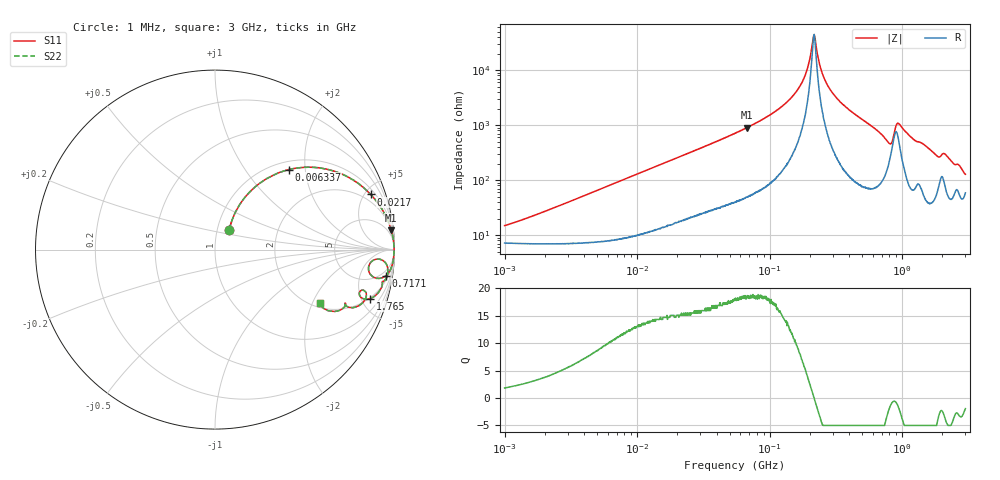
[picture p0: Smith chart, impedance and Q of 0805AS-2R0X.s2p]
!s-Parameter Generated by FASTRON Sdn. Bhd.
!FASTRON P/N : 0805AS-2R0X
!Keysight Technologies: E4991B_MY54100416_A.01.15
!Date: Mon Jun 15 12:57:28 2026
!Version  :Rev01  Mon Jun 15 12:57:28 2026
!Data & Calibration Information:
!Freq  S11  S21  S12  S22
!PortZ  Port1:50+j0  Port2:50+j0
!When reading reference impedance value at option line is always used.
! Remarks : This data is being provided solely for informational purposes.
# Hz S dB R 50
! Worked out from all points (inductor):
!   1601 points, 1 MHz to 3 GHz, reference 50 ohm
!   read as one part in series: L = 2.06 uH near 1.617 MHz
!   highest Q = 18.5 at 67.25 MHz (marker M1), where L = 2.13 uH
!   self-resonance near 215.8 MHz
!   S11 on the Smith chart (normalised r, x): 1 MHz: 1.14, +0.26; 6.337 MHz: 1.16, +1.64; 21.7 MHz: 1.36, +5.49; 717.1 MHz: 3, -13; 1.765 GHz: 1.91, -5.90; 3 GHz: 2.17, -2.27
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1000000  -17.20 54.2  -0.66 -6.9  -0.66 -6.9  -17.20 54.2
3804036  -7.49 57.0  -1.43 -24.7  -1.43 -24.7  -7.49 57.0
6337400  -4.34 47.3  -2.64 -37.2  -2.64 -37.2  -4.34 47.3
1.447069e7  -1.36 27.4  -6.71 -58.6  -6.71 -58.6  -1.36 27.4
2.170294e7  -0.72 19.5  -9.53 -66.7  -9.53 -66.7  -0.72 19.5
5.504702e7  -0.15 7.9  -17.20 -78.9  -17.20 -78.9  -0.15 7.9
6.724529e7  -0.10 6.3  -19.20 -80.6  -19.20 -80.6  -0.10 6.3
1.114693e8  -0.04 3.1  -25.20 -83.5  -25.20 -83.5  -0.04 3.1
1.543168e8  -0.03 1.5  -31.40 -82.9  -31.40 -82.9  -0.03 1.5
1.857042e8  -0.02 0.7  -38.20 -78.5  -38.20 -78.5  -0.02 0.7
1.971969e8  -0.02 0.4  -42.40 -71.9  -42.40 -71.9  -0.02 0.4
2.083556e8  -0.02 0.2  -48.50 -52.7  -48.50 -52.7  -0.02 0.2
2.19047e8  -0.02 -0.1  -52.10 23.1  -52.10 23.1  -0.02 -0.1
2.507343e8  -0.02 -0.7  -38.60 77.9  -38.60 77.9  -0.02 -0.7
3.062963e8  -0.03 -1.6  -31.00 83.2  -31.00 83.2  -0.03 -1.6
7.171101e8  -0.32 -8.6  -16.40 72.2  -16.40 72.2  -0.32 -8.6
7.925923e8  -0.87 -10.0  -14.40 55.3  -14.40 55.3  -0.87 -10.0
9.395906e8  -0.42 -4.4  -21.00 55.4  -21.00 55.4  -0.42 -4.4
1.194682e9  -0.29 -9.6  -15.50 73.8  -15.50 73.8  -0.29 -9.6
1.76507e9  -0.84 -17.5  -10.40 63.7  -10.40 63.7  -0.84 -17.5
2.071593e9  -1.16 -15.9  -10.80 56.5  -10.80 56.5  -1.16 -15.9
3e9  -3.67 -27.1  -5.81 35.7  -5.81 35.7  -3.67 -27.1
